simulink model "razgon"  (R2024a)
settings: Solver=VariableStepAuto  StartTime=0.0  StopTime=1000  MaxStep=1e-3  RelTol=1e-10  AbsTol=1e-10
undefined symbols (not defined in the file or in its folder): cx, deltaP, Flob, fsh, g, irk, kpdt, ksN, kv, M_kr, Ma, n_kr, num_per, rk0, row, sigma1_c, sigma2, tper, ugp, ukp, ukr, urk, v0

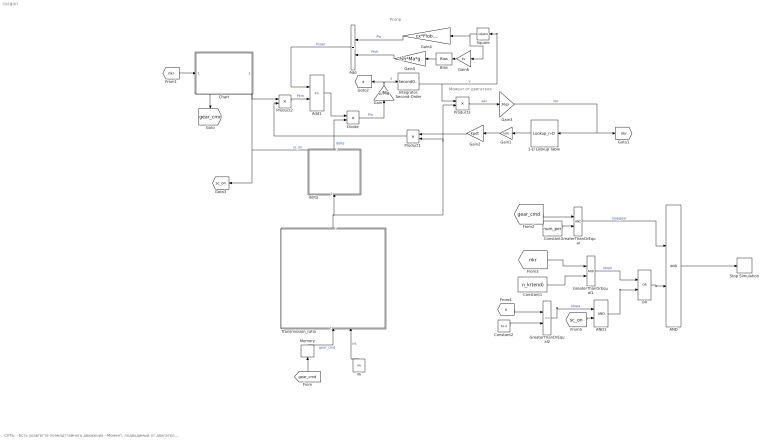
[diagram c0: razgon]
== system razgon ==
  note: Момент от двигателя
  note: СУТЬ: - Есть уоавгегте поямлдтгейного движения - Момент, подводимый от двигателя, задаётся частотой и ВСХ двигателя (частота считается из скорости движения) - Передача выбирается по макс. оборотам - Передаточное число трансмиссии выбирается по выбранной передаче - Коэффициент учет вращающихся масс выбирается по передаче и вкл/выкл "сцеплению" (сцепления в этой модели нет, просто момент от двигателя во время переключения не передается) - Время симуляции - 1000 секунд, НО она останавливается, когда либо включена последняя передача и обороты максимальные, либо когда на текущей (не последней) передаче устанавливается постоянная скорость
  note: Pсопр
  1-D Lookup Table : Lookup_n-D  NumberOfTableDimensions=1  BreakpointsForDimension1=n_kr  Table=M_kr  InternalRulePriority=Speed  RndMeth=Simplest
  AND : Logic  IconShape=distinctive  AllPortsSameDT=off  OutDataTypeStr=boolean
  AND1 : Logic  IconShape=distinctive  AllPortsSameDT=off  OutDataTypeStr=boolean
  Add : Sum
  Add1 : Sum  Inputs=-+
  Bias : Bias  Bias=1
  Chart : Stateflow chart  TreatAsAtomicUnit=on
  Constant : Constant  Value=num_per
  Constant1 : Constant  Value=n_kr(end)
  Constant2 : Constant  Value=1e-2
  Divide : Product  Inputs=*/
  Gain : Gain  Gain=1/Ma
  Gain1 : Gain  Gain=ksN
  Gain2 : Gain  Gain=kpdt
  Gain3 : Gain  Gain=30/pi
  Gain4 : Gain  Gain=cx*Flob*row*0.5
  Gain5 : Gain  Gain=fsh*Ma*g
  Gain6 : Gain  Gain=kv
  GreaterThanOrEqual : RelationalOperator  OutDataTypeStr=boolean  RndMeth=Simplest
  GreaterThanOrEqual1 : RelationalOperator  OutDataTypeStr=boolean  RndMeth=Simplest
  GreaterThanOrEqual2 : RelationalOperator  Operator=<=  OutDataTypeStr=boolean  RndMeth=Simplest
  "Integrator, Second-Order" : SecondOrderIntegrator  ICDXDT=v0+1e-3
  Memory : Memory  InitialCondition=1
  OR : Logic  Operator=OR  IconShape=distinctive  AllPortsSameDT=off  OutDataTypeStr=boolean
  Product1 : Product
  Product2 : Product
  Product3 : Product
  Square : Math  Operator=square
  Stop Simulation : Stop
  Transmission_ratio : Subsystem
  delta : Subsystem
  irk : Constant  Value=irk
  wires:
  "Integrator, Second-Order"/2 -> Product3/1, Square/1  "v"
  Product3/1 -> Gain3/1  "wkr"
  Gain1/1 -> Gain2/1
  Square/1 -> Gain6/1, Gain4/1
  1-D Lookup Table/1 -> Gain1/1
  Gain2/1 -> Product1/1
  Gain4/1 -> Add/1  "Pw"
  Product1/1 -> Product2/2
  Bias/1 -> Gain5/1
  Gain6/1 -> Bias/1
  Gain5/1 -> Add/2  "Pfsh"
  Add/1 -> Add1/1  "Psopr"
  Product2/1 -> Add1/2  "Pkm"
  Divide/1 -> Gain/1  "Pin"
  Add1/1 -> Divide/1
  Transmission_ratio/1(utr/rk0) -> Product3/2, Product1/2, delta/1(In1)
  irk/1 -> Transmission_ratio/2(irk)  "irk"
  delta/1(Out1) -> Divide/2  "delta"
  Chart/1(sc_on) -> Product2/1, [sc_on], delta/2(sc_on)  "sc_on"
  Chart/2(current_gear) -> [gear_cmd]
  [gear_cmd] -> Memory/1
  [nkr] -> Chart/1(n)
  "Integrator, Second-Order"/1 -> ?  "x"
  Memory/1 -> Transmission_ratio/1(ikp)  "gear_cmd"
  Gain3/1 -> [nkr], 1-D Lookup Table/1  "nkr"
  Gain/1 -> "Integrator, Second-Order"/1, [a]  "a"
  Constant/1 -> GreaterThanOrEqual/2
  [gear_cmd] -> GreaterThanOrEqual/1
  Constant1/1 -> GreaterThanOrEqual1/2
  [nkr] -> GreaterThanOrEqual1/1
  GreaterThanOrEqual/1 -> AND/1  "stopgear"
  GreaterThanOrEqual1/1 -> OR/1  "stopn"
  AND/1 -> Stop Simulation/1
  [a] -> GreaterThanOrEqual2/1
  Constant2/1 -> GreaterThanOrEqual2/2
  GreaterThanOrEqual2/1 -> AND1/1  "stopa"
  OR/1 -> AND/2
  [sc_on] -> AND1/2
  AND1/1 -> OR/2

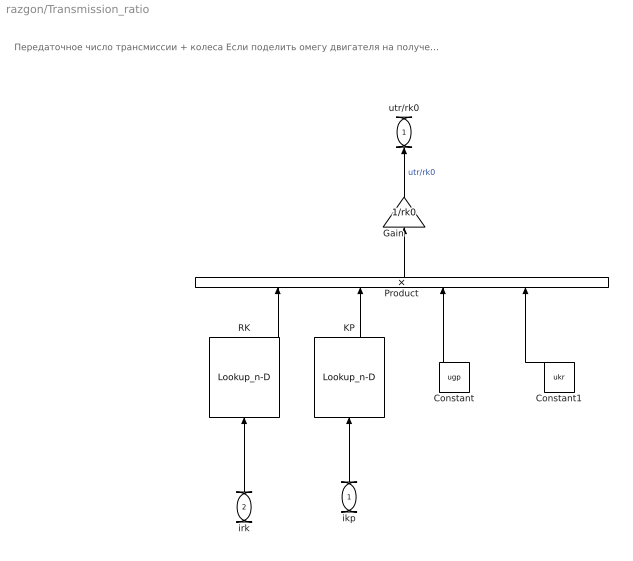
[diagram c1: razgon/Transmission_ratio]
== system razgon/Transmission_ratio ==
  note: Передаточное число трансмиссии + колеса Если поделить омегу двигателя на полученное число, получим скорость машины
  ikp : Inport
  irk : Inport  Port=2
  Constant : Constant  Value=ugp
  Constant1 : Constant  Value=ukr
  Gain : Gain  Gain=1/rk0
  KP : Lookup_n-D  NumberOfTableDimensions=1  BreakpointsForDimension1=1:length(ukp)  Table=ukp  InterpMethod=Flat  InternalRulePriority=Speed  RndMeth=Simplest
  Product : Product  Inputs=4
  RK : Lookup_n-D  NumberOfTableDimensions=1  BreakpointsForDimension1=0:length(urk)  Table=[urk(1) urk]  InterpMethod=Flat  InternalRulePriority=Speed  RndMeth=Simplest
  utr/rk0 : Outport
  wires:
  ikp/1 -> KP/1
  Constant/1 -> Product/3
  Product/1 -> Gain/1
  irk/1 -> RK/1
  RK/1 -> Product/1
  KP/1 -> Product/2
  Constant1/1 -> Product/4
  Gain/1 -> utr/rk0/1  "utr/rk0"

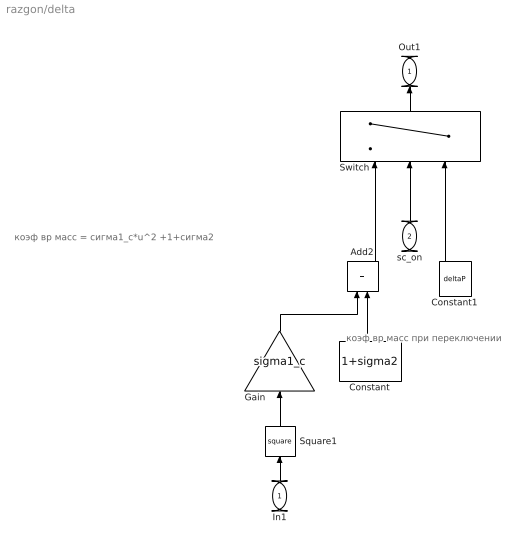
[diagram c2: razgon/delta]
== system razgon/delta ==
  note: коэф вр масс = сигма1_с*u^2 +1+сигма2
  note: коэф вр масс при переключении
  In1 : Inport
  sc_on : Inport  Port=2
  Add2 : Sum
  Constant : Constant  Value=1+sigma2
  Constant1 : Constant  Value=deltaP
  Gain : Gain  Gain=sigma1_c
  Square1 : Math  Operator=square
  Switch : Switch  Criteria=u2 > Threshold
  Out1 : Outport
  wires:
  In1/1 -> Square1/1
  Gain/1 -> Add2/1
  Square1/1 -> Gain/1
  Constant/1 -> Add2/2
  Add2/1 -> Switch/1
  Switch/1 -> Out1/1
  Constant1/1 -> Switch/3
  sc_on/1 -> Switch/2

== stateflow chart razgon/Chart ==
  state Running
    en:sc_on=1;
  state Gear_UP
    en: sc_on=0;
    current_gear=current_gear+1;
  state <!DOCTYPE HTML PUBLIC "-//W3C//DTD HTML 4.0//EN" "http://www.w3.org/TR/REC-html40/strict.dtd"> [group]
    <html><head><meta name="qrichtext" content="1" /><style type="text/css">
    p, li { white-space: pre-wrap; }
    </style></head><body align="left" style=" font-family:'Helvetica'; font-size:12px; font-weight:400; font-style:normal;">
    <ol style="margin-top: 0px; margin-bottom: 0px; margin-left: 0px; margin-right: 0px; -qt-list-indent: 1;"><li align="left" style=" margin-top:0px; margin-bottom:0px; margin-left:9px; margin-right:0px; -qt-block-indent:0; text-indent:0px;">Если обороты большие - перейти в состояние переключения передачи</li>
    <li align="left" style=" margin-top:0px; margin-bottom:0px; margin-left:9px; margin-right:0px; -qt-block-indent:0; text-indent:0px;">... И повысить передачу</li>
    <li align="left" style=" margin-top:0px; margin-bottom:0px; margin-left:9px; margin-right:0px; -qt-block-indent:0; text-indent:0px;">Подождать время переключения</li>
    <li align="left" style=" margin-top:0px; margin-bottom:0px; margin-left:9px; margin-right:0px; -qt-block-indent:0; text-indent:0px;">Вернуться в состояние Running (включенное сцепление)</li></ol></body></html>
  (default) -> Running : {current_gear=1;}
  Running -> Gear_UP : [n>n_kr(end)-10 && current_gear<num_per]
  Gear_UP -> Running : [after(tper,sec)]
  data: sc_on output; tper parameter; current_gear output; n input; num_per parameter; n_kr parameter
